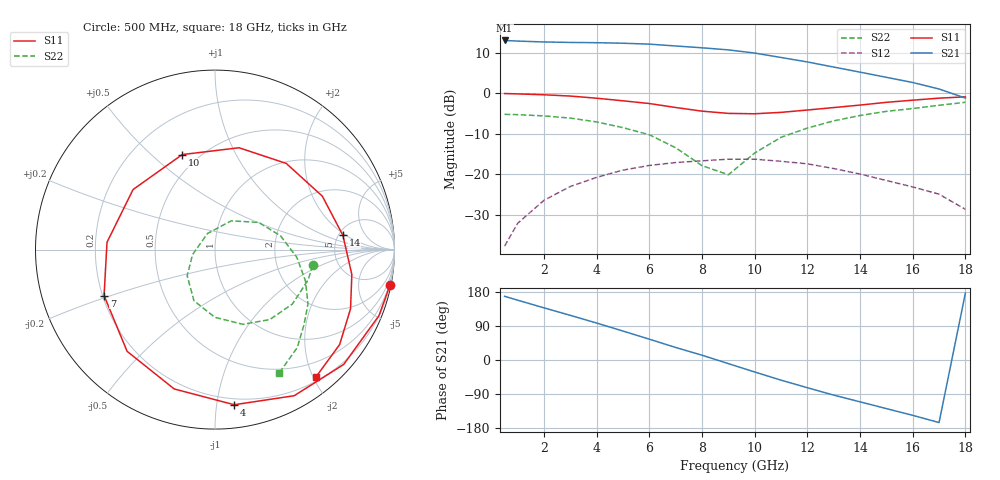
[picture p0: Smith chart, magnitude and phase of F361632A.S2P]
!ATF-36163
!2V 10mA
! last updated 11-10-95
# ghz s ma r 50
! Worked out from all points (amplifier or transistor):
!   19 points, 500 MHz to 18 GHz, reference 50 ohm
!   highest |S21| = 13.1 dB at 500 MHz (marker M1)
!   |S21| within 3 dB of that: start of sweep to 9.856 GHz
!   unconditionally stable (mu >= 1): 10.96 GHz to end of sweep
!   at 3 GHz: K = 0.32, MSG = 17.8 dB, |S12| = -23.0 dB
!   at 9 GHz: K = 0.85, MSG = 13.5 dB, |S12| = -16.2 dB
!   at 18 GHz: K = 1.64, MAG = 9.1 dB, |S12| = -28.6 dB
!   lowest NFmin = 0.46 dB at 2 GHz
!   S11 on the Smith chart (normalised r, x): 500 MHz: 0, -10; 4 GHz: 0.16, -1.12; 7 GHz: 0.21, -0.19; 10 GHz: 0.41, +0.63; 14 GHz: 5.47, +1.78; 18 GHz: 0.26, -2.04
0.5  0.995 -11.4  4.499 168.1  0.013 79.4  0.551 -9.1
1  0.985 -21.9  4.418 157.7  0.025 71.2  0.546 -18.0
2  0.961 -41.7  4.31 137.5  0.048 55.5  0.527 -35.2
3  0.926 -61.5  4.252 117.7  0.071 39.9  0.495 -52.0
4  0.871 -82.9  4.221 97.5  0.092 23.3  0.444 -69.6
5  0.809 -106.3  4.157 76.3  0.113 5.7  0.377 -90.2
6  0.749 -130.8  4.052 54.9  0.129 -11.6  0.308 -112.4
7  0.669 -157.5  3.844 33.0  0.14 -29.9  0.213 -136.6
8  0.603 176.1  3.651 12.6  0.147 -44.1  0.128 -167.6
9  0.566 143.8  3.441 -9.6  0.154 -59.8  0.099 115.0
10  0.56 109.0  3.144 -31.7  0.154 -75.8  0.184 60.6
11  0.583 76.7  2.772 -53.2  0.145 -91.0  0.287 31.9
12  0.623 50.4  2.441 -73.2  0.135 -104.2  0.373 11.9
13  0.668 26.5  2.112 -92.7  0.118 -116.9  0.458 -5.4
14  0.717 6.3  1.828 -110.4  0.101 -125.8  0.533 -19.0
15  0.775 -10.3  1.577 -128.3  0.084 -134.3  0.6 -30.3
16  0.824 -23.6  1.362 -146.0  0.07 -139.2  0.65 -40.3
17  0.873 -37.3  1.132 -165.1  0.057 -146.7  0.713 -50.0
18  0.906 -51.7  0.875 176.7  0.037 -153.1  0.776 -62.7
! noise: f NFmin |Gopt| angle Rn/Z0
2  0.46  0.84  27.73  0.376
3  0.5  0.761  40.84  0.311
5  0.59  0.605  70.44  0.197
7  0.68  0.486  103.1  0.116
9  0.8  0.332  135  0.074
10  0.86  0.229  164.9  0.07
12  1.02  0.183  -93.33  0.124
14  1.22  0.344  -16.37  0.304
16  1.51  0.575  18.96  0.569
18  1.92  0.657  50.21  1.096
